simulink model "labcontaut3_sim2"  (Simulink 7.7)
settings: Solver=ode45  StartTime=0.0  StopTime=10.0  RelTol=1e-3

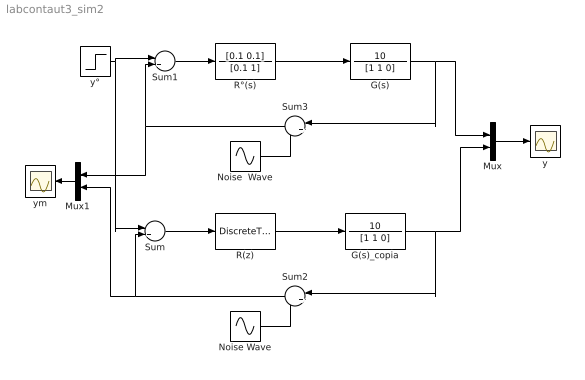
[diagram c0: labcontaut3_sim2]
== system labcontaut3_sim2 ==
  G(s) : TransferFcn  Numerator=10  Denominator=[1 1 0]
  G(s)_copia : TransferFcn  Numerator=10  Denominator=[1 1 0]
  Mux : Mux  Inputs=2
  Mux1 : Mux  Inputs=2
  Noise  Wave : Sin  Amplitude=0.05  Frequency=500  SampleTime=0
  Noise Wave : Sin  Amplitude=0.05  Frequency=500  SampleTime=0
  R(z) : DiscreteTransferFcn  Numerator=[1.1 -1]  Denominator=[2 -1]  SampleTime=0.1
  R°(s) : TransferFcn  Numerator=[0.1 0.1]  Denominator=[0.1 1]
  Sum : Sum  Inputs=|+-
  Sum1 : Sum  Inputs=|+-
  Sum2 : Sum  Inputs=|++
  Sum3 : Sum  Inputs=|++
  y : Scope
  ym : Scope
  y° : Step  Time=0  SampleTime=0
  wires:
  Sum1/1 -> R°(s)/1
  y°/1 -> Sum1/1, Sum/1
  G(s)/1 -> Mux/1, Sum3/1
  Mux/1 -> y/1
  R°(s)/1 -> G(s)/1
  Sum/1 -> R(z)/1
  G(s)_copia/1 -> Mux/2, Sum2/1
  R(z)/1 -> G(s)_copia/1
  Sum2/1 -> Sum/2, Mux1/2
  Noise Wave/1 -> Sum2/2
  Sum3/1 -> Sum1/2, Mux1/1
  Noise  Wave/1 -> Sum3/2
  Mux1/1 -> ym/1
